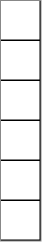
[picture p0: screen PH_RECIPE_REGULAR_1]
VISUALIZATION PH_RECIPE_REGULAR_1  // 42x242
VAR_IN_OUT
	RECIPE_CTRL_V2 : ST_RecipeCtrl_2;
END_VAR
    Frame (0,0 40x40)
        shows PH_RECIPE_PAGE_TOP_2(RECIPE_CTRL_V2 := RECIPE_CTRL_V2)
        pReferences[0]: m_Input_RECIPE_CTRL_V2=m_Input_RECIPE_CTRL_V2
    Frame (0,40 40x40)
        shows PH_RECIPE_PAGE_UP_2(RECIPE_CTRL_V2 := RECIPE_CTRL_V2)
        pReferences[0]: m_Input_RECIPE_CTRL_V2=m_Input_RECIPE_CTRL_V2
    Frame (0,80 40x40)
        shows PH_RECIPE_SCROLL_UP_2(RECIPE_CTRL_V2 := RECIPE_CTRL_V2)
        pReferences[0]: m_Input_RECIPE_CTRL_V2=m_Input_RECIPE_CTRL_V2
    Frame (0,120 40x40)
        shows PH_RECIPE_SCROLL_DOWN_2(RECIPE_CTRL_V2 := RECIPE_CTRL_V2)
        pReferences[0]: m_Input_RECIPE_CTRL_V2=m_Input_RECIPE_CTRL_V2
        p2738717112: RECIPE_CTRL_V2.sStatus.i16RegularOffset
    Rectangle (0,40 40x40)
        tap RECIPE_CTRL_V2.sCmd.bPageUp
    Polygon (20,60), colour toggle: (RECIPE_CTRL_V2.sCmd.bPageUp) <> 0
        tap RECIPE_CTRL_V2.sCmd.bPageUp
    Polygon (20,50), colour toggle: (RECIPE_CTRL_V2.sCmd.bPageUp) <> 0
        tap RECIPE_CTRL_V2.sCmd.bPageUp
    Rectangle (0,0 40x40)
        tap RECIPE_CTRL_V2.sCmd.bJumpTop
    Polyline (35,10), colour toggle: (RECIPE_CTRL_V2.sCmd.bJumpTop) <> 0
        tap RECIPE_CTRL_V2.sCmd.bJumpTop
    Polygon (20,20), colour toggle: (RECIPE_CTRL_V2.sCmd.bJumpTop) <> 0
        tap RECIPE_CTRL_V2.sCmd.bJumpTop
    Polygon (20,10), colour toggle: (RECIPE_CTRL_V2.sCmd.bJumpTop) <> 0
        tap RECIPE_CTRL_V2.sCmd.bJumpTop
    Rectangle (0,80 40x40)
        tap RECIPE_CTRL_V2.sCmd.bScrollUp
    Polygon (20,90), colour toggle: (RECIPE_CTRL_V2.sCmd.bScrollUp) <> 0
        tap RECIPE_CTRL_V2.sCmd.bScrollUp
    Rectangle (0,120 40x40)
        p2738717112: RECIPE_CTRL_V2.sStatus.i16RegularOffset
        tap RECIPE_CTRL_V2.sCmd.bScrollDown
    Polygon (20,150), colour toggle: (RECIPE_CTRL_V2.sCmd.bScrollDown) <> 0
        p2738717112: RECIPE_CTRL_V2.sStatus.i16RegularOffset
        tap RECIPE_CTRL_V2.sCmd.bScrollDown
    Rectangle (0,160 40x40)
        p2738717112: RECIPE_CTRL_V2.sStatus.i16RegularOffset
        tap RECIPE_CTRL_V2.sCmd.bPageDown
    Polygon (20,180), colour toggle: (RECIPE_CTRL_V2.sCmd.bPageDown) <> 0
        p2738717112: RECIPE_CTRL_V2.sStatus.i16RegularOffset
        tap RECIPE_CTRL_V2.sCmd.bPageDown
    Polygon (20,190), colour toggle: (RECIPE_CTRL_V2.sCmd.bPageDown) <> 0
        p2738717112: RECIPE_CTRL_V2.sStatus.i16RegularOffset
        tap RECIPE_CTRL_V2.sCmd.bPageDown
    Rectangle (0,200 40x40)
        p2738717112: RECIPE_CTRL_V2.sStatus.i16RegularOffset
        tap RECIPE_CTRL_V2.sCmd.bJumpBottom
    Polyline (35,230), colour toggle: (RECIPE_CTRL_V2.sCmd.bJumpBottom) <> 0
        p2738717112: RECIPE_CTRL_V2.sStatus.i16RegularOffset
        tap RECIPE_CTRL_V2.sCmd.bJumpBottom
    Polygon (20,220), colour toggle: (RECIPE_CTRL_V2.sCmd.bJumpBottom) <> 0
        p2738717112: RECIPE_CTRL_V2.sStatus.i16RegularOffset
        tap RECIPE_CTRL_V2.sCmd.bJumpBottom
    Polygon (20,230), colour toggle: (RECIPE_CTRL_V2.sCmd.bJumpBottom) <> 0
        p2738717112: RECIPE_CTRL_V2.sStatus.i16RegularOffset
        tap RECIPE_CTRL_V2.sCmd.bJumpBottom
    Rectangle (0,120 40x0)
        p1126004900: RECIPE_CTRL_V2.sStatus.i16RegularOffset
END_VISUALIZATION
